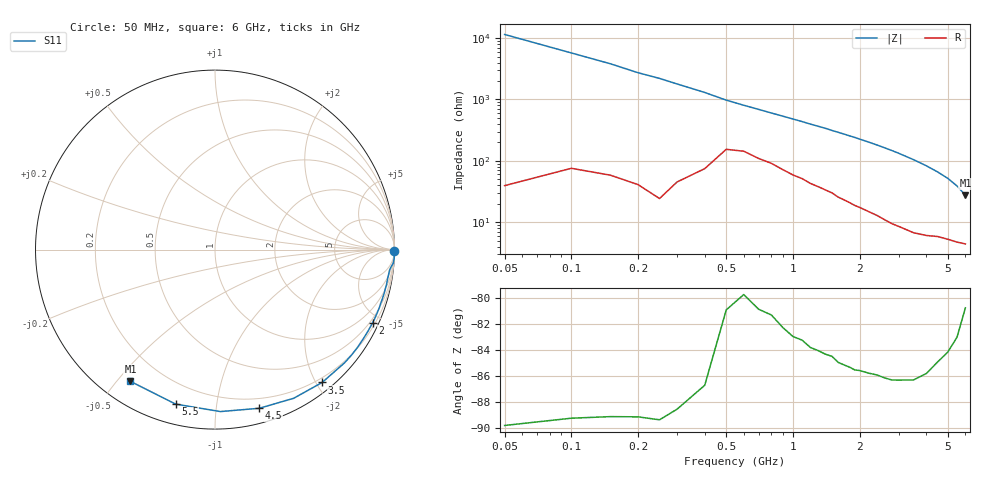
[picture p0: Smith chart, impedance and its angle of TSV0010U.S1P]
! SIEMENS Small Signal Semiconductors
! BAT14-03W
! Si Schottky Diode in SOD323
! IF = 0.01 mA
! S-Parameters:  November  1995
# GHz  S  MA  R  50
!  f  S11
! GHz  MAG  ANG
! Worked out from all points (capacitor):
!   34 points, 50 MHz to 6 GHz, reference 50 ohm
!   read as one part to ground: C = 278 fF near 50 MHz
!   lowest |Z| = 27.5 ohm at 6 GHz (marker M1)
!   S11 on the Smith chart (normalised r, x): 50 MHz: open; 2 GHz: 0.35, -4.50; 3.5 GHz: 0.13, -2.08; 4.5 GHz: 0.12, -1.31; 5.5 GHz: 0.09, -0.77; 6 GHz: 0.09, -0.54
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0.05  1 -0.5
0.15  0.9996 -1.5
0.2  0.9994 -2.1
0.25  0.9995 -2.6
0.4  0.9956 -4.4
0.5  0.984 -5.8
0.6  0.9782 -7.0
0.7  0.9773 -8.2
0.8  0.9754 -9.4
1  0.9751 -11.8
1.1  0.9737 -13.0
1.2  0.9736 -14.3
1.4  0.9718 -16.7
1.5  0.9705 -18.1
1.6  0.9711 -19.4
1.9  0.9694 -23.4
2  0.968 -24.9
2.2  0.9662 -27.8
2.4  0.9641 -30.9
2.6  0.9629 -34.2
2.8  0.9614 -37.6
3  0.9585 -41.2
3.5  0.951 -51.1
4  0.9373 -62.1
4.5  0.9179 -74.4
5  0.9029 -88.1
5.5  0.8883 -104.3
6  0.8723 -122.7
